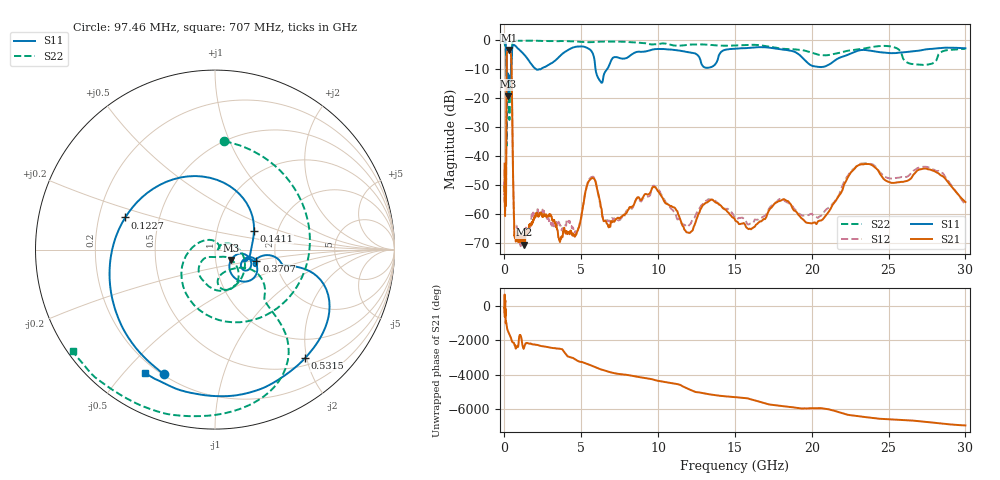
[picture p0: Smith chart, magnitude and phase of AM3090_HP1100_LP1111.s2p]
! Date/Time: Thu, Feb 28, 2019 2:07 PM
! Network Analyzer: Agilent Technologies E8364B Rev: A.07.50.67
! Sweep from 0.010 to 30.000 GHz, 1601 Points, Sweep Type: LOG
! Power Supply: 5.022 V, 0.002 A
# Hz S DB R 50
!freq MagS11 AngS11 MagS21 AngS21 MagS12 AngS12 MagS22 AngS22
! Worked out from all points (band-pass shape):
!   1601 points, 10 MHz to 30 GHz, reference 50 ohm
!   highest |S21| = -3.50 dB at 302 MHz (marker M1); lowest = -70.5 dB at 1.263 GHz (marker M2)
!   |S21| within 3 dB of the highest: 145.2 MHz to 443.1 MHz (297.8 MHz wide, 101 % of centre)
!   lowest |S11| = -19.4 dB at 249.7 MHz (marker M3), VSWR 1.24, Z = 59.4 - j6.93 ohm
!   |S11| at or under -10 dB: 136.1 MHz to 430.7 MHz (294.6 MHz wide, 104 % of centre); 2.033 GHz to 2.388 GHz (354.6 MHz wide, 16 % of centre); 5.925 GHz to 6.695 GHz (770 MHz wide, 12.2 % of centre)
!   |S22| runs from -36.4 to -0.2 dB; largest |S21 - S12| = 0.0096
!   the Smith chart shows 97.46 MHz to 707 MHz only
!   S11 on the Smith chart (normalised r, x): 97.46 MHz: 0.20, -0.65; 122.7 MHz: 0.31, +0.16; 141.1 MHz: 1.51, +0.34; 370.7 MHz: 1.58, -0.21; 531.5 MHz: 0.62, -1.96; 707 MHz: 0.16, -0.57
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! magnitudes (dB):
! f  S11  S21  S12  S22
! 10 MHz  -0.2  -42.6  -51.0  -0.7
! 38.04 MHz  -0.4  -58.4  -58.9  -1.6
! 48.61 MHz  -0.6  -48.1  -49.5  -1.8
! 97.46 MHz  -2.5  -56.1  -55.6  -4.4
! 122.7 MHz  -5.5  -29.8  -29.8  -6.3
! 141.1 MHz  -12.3  -7.9  -7.8  -23.0
! 144.7 MHz  -13.4  -6.6  -6.6  -28.3
! 249.7 MHz  -19.4  -3.5  -3.5  -13.9
! 302 MHz  -13.2  -3.5  -3.5  -19.2
! 370.7 MHz  -12.4  -4.1  -4.1  -12.6
! 457.4 MHz  -7.9  -8.1  -8.1  -7.6
! 531.5 MHz  -2.1  -37.0  -37.0  -0.7
! 550.5 MHz  -1.9  -43.8  -43.5  -0.5
! 707 MHz  -2.0  -67.2  -68.2  -0.2
! 1.263 GHz  -5.0  -70.5  -67.0  -0.3
! 2.084 GHz  -10.2  -60.0  -59.8  -0.3
! 4.571 GHz  -2.5  -67.7  -65.4  -0.5
! 5.697 GHz  -4.2  -47.6  -47.2  -0.8
! 7.926 GHz  -6.3  -59.6  -59.0  -0.7
! 20.1 GHz  -9.1  -62.9  -60.5  -4.6
! 23.48 GHz  -3.5  -42.7  -42.5  -2.9
! 30 GHz  -2.9  -55.8  -56.7  -3.1
